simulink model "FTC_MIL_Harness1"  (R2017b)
settings: Solver=FixedStepDiscrete  StartTime=0.0  StopTime=4  FixedStep=0.01  RelTol=1e-3  EnableMultiTasking=on
undefined symbols (not defined in the file): sigbuilder_block

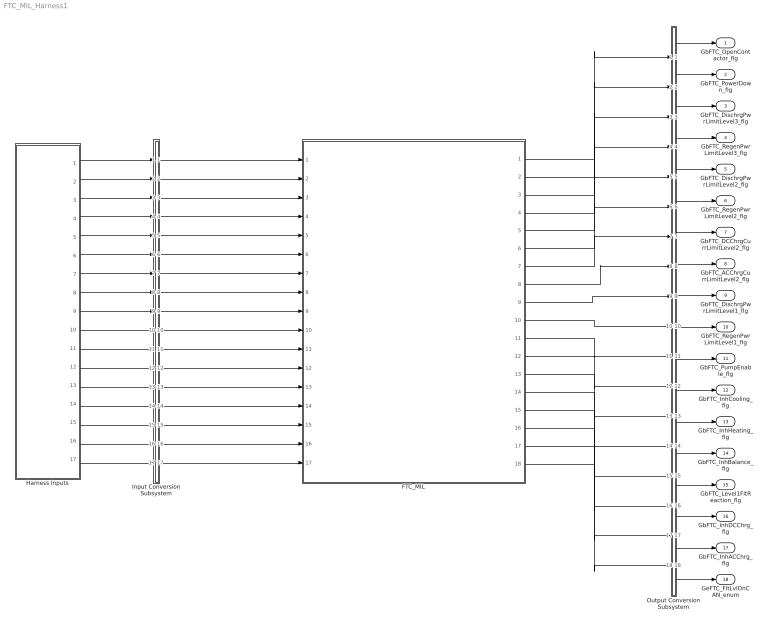
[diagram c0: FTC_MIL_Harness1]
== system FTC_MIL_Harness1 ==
  FTC_MIL : ModelReference  ModelNameDialog=FTC_MIL  SimulationMode=Normal  ModelReferenceVersion='M102C103'
  Harness Inputs : Subsystem  Tag=STV Subsys  LoadFcn=sigbuilder_block('load');  StartFcn=sigbuilder_block('start');  StopFcn=sigbuilder_block('stop');  ClipboardFcn=sigbuilder_block('clipboard');  mask(Sigbuilder block){tuvar=[0:10]}
      mask init:
      | if ~strcmp(get_param(bdroot(gcb),'SimulationStatus'),'stopped'),tuvar = sigbuilder_block('maskInit'); end
  Input Conversion Subsystem : Subsystem  Tag=__SLT_ICS__  Description=Signal spec. and routing
  Output Conversion Subsystem : Subsystem  Tag=__SLT_OCS__  Description=Signal spec. and routing
  GbFTC_OpenContactor_flg : Outport  OutDataTypeStr=boolean  PortDimensions=[1]
  GbFTC_PowerDown_flg : Outport  Port=2  OutDataTypeStr=boolean  PortDimensions=[1]
  GbFTC_DischrgPwrLimitLevel3_flg : Outport  Port=3  OutDataTypeStr=boolean  PortDimensions=[1]
  GbFTC_RegenPwrLimitLevel3_flg : Outport  Port=4  OutDataTypeStr=boolean  PortDimensions=[1]
  GbFTC_DischrgPwrLimitLevel2_flg : Outport  Port=5  OutDataTypeStr=boolean  PortDimensions=[1]
  GbFTC_RegenPwrLimitLevel2_flg : Outport  Port=6  OutDataTypeStr=boolean  PortDimensions=[1]
  GbFTC_DCChrgCurrLimitLevel2_flg : Outport  Port=7  OutDataTypeStr=boolean  PortDimensions=[1]
  GbFTC_ACChrgCurrLimitLevel2_flg : Outport  Port=8  OutDataTypeStr=boolean  PortDimensions=[1]
  GbFTC_DischrgPwrLimitLevel1_flg : Outport  Port=9  OutDataTypeStr=boolean  PortDimensions=[1]
  GbFTC_RegenPwrLimitLevel1_flg : Outport  Port=10  OutDataTypeStr=boolean  PortDimensions=[1]
  GbFTC_PumpEnable_flg : Outport  Port=11  OutDataTypeStr=boolean  PortDimensions=[1]
  GbFTC_InhCooling_flg : Outport  Port=12  OutDataTypeStr=boolean  PortDimensions=[1]
  GbFTC_InhHeating_flg : Outport  Port=13  OutDataTypeStr=boolean  PortDimensions=[1]
  GbFTC_InhBalance_flg : Outport  Port=14  OutDataTypeStr=boolean  PortDimensions=[1]
  GbFTC_Level1FltReaction_flg : Outport  Port=15  OutDataTypeStr=boolean  PortDimensions=[1]
  GbFTC_InhDCChrg_flg : Outport  Port=16  OutDataTypeStr=boolean  PortDimensions=[1]
  GbFTC_InhACChrg_flg : Outport  Port=17  OutDataTypeStr=boolean  PortDimensions=[1]
  GeFTC_FltLvlOnCAN_enum : Outport  Port=18  OutDataTypeStr=uint8  PortDimensions=[1]
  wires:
  Harness Inputs/1(GbISP_OpenContactor_flg) -> Input Conversion Subsystem/1(Inport_1)
  Harness Inputs/2(GbISP_PowerDown_flg) -> Input Conversion Subsystem/2(Inport_2)
  Harness Inputs/3(GbISP_DischrgPwrLimitLevel3_flg) -> Input Conversion Subsystem/3(Inport_3)
  Harness Inputs/4(GbISP_RegenPwrLimitLevel3_flg) -> Input Conversion Subsystem/4(Inport_4)
  Harness Inputs/5(GbISP_DischrgPwrLimitLevel2_flg) -> Input Conversion Subsystem/5(Inport_5)
  Harness Inputs/6(GbISP_RegenPwrLimitLevel2_flg) -> Input Conversion Subsystem/6(Inport_6)
  Harness Inputs/7(GbISP_DCChrgCurrLimitLevel2_flg) -> Input Conversion Subsystem/7(Inport_7)
  Harness Inputs/8(GbISP_ACChrgCurrLimitLevel2_flg) -> Input Conversion Subsystem/8(Inport_8)
  Harness Inputs/9(GbISP_DischrgPwrLimitLevel1_flg) -> Input Conversion Subsystem/9(Inport_9)
  Harness Inputs/10(GbISP_RegenPwrLimitLevel1_flg) -> Input Conversion Subsystem/10(Inport_10)
  Harness Inputs/11(GbISP_PumpEnable_flg) -> Input Conversion Subsystem/11(Inport_11)
  Harness Inputs/12(GbISP_InhCooling_flg) -> Input Conversion Subsystem/12(Inport_12)
  Harness Inputs/13(GbISP_InhHeating_flg) -> Input Conversion Subsystem/13(Inport_13)
  Harness Inputs/14(GbISP_InhBalance_flg) -> Input Conversion Subsystem/14(Inport_14)
  Harness Inputs/15(GbISP_FltReactionReserved_flg) -> Input Conversion Subsystem/15(Inport_15)
  Harness Inputs/16(GbISP_InhDCChrg_flg) -> Input Conversion Subsystem/16(Inport_16)
  Harness Inputs/17(GbISP_InhACChrg_flg) -> Input Conversion Subsystem/17(Inport_17)
  Output Conversion Subsystem/1(Outport_1) -> GbFTC_OpenContactor_flg/1
  Output Conversion Subsystem/2(Outport_2) -> GbFTC_PowerDown_flg/1
  Output Conversion Subsystem/3(Outport_3) -> GbFTC_DischrgPwrLimitLevel3_flg/1
  Output Conversion Subsystem/4(Outport_4) -> GbFTC_RegenPwrLimitLevel3_flg/1
  Output Conversion Subsystem/5(Outport_5) -> GbFTC_DischrgPwrLimitLevel2_flg/1
  Output Conversion Subsystem/6(Outport_6) -> GbFTC_RegenPwrLimitLevel2_flg/1
  Output Conversion Subsystem/7(Outport_7) -> GbFTC_DCChrgCurrLimitLevel2_flg/1
  Output Conversion Subsystem/8(Outport_8) -> GbFTC_ACChrgCurrLimitLevel2_flg/1
  Output Conversion Subsystem/9(Outport_9) -> GbFTC_DischrgPwrLimitLevel1_flg/1
  Output Conversion Subsystem/10(Outport_10) -> GbFTC_RegenPwrLimitLevel1_flg/1
  Output Conversion Subsystem/11(Outport_11) -> GbFTC_PumpEnable_flg/1
  Output Conversion Subsystem/12(Outport_12) -> GbFTC_InhCooling_flg/1
  Output Conversion Subsystem/13(Outport_13) -> GbFTC_InhHeating_flg/1
  Output Conversion Subsystem/14(Outport_14) -> GbFTC_InhBalance_flg/1
  Output Conversion Subsystem/15(Outport_15) -> GbFTC_Level1FltReaction_flg/1
  Output Conversion Subsystem/16(Outport_16) -> GbFTC_InhDCChrg_flg/1
  Output Conversion Subsystem/17(Outport_17) -> GbFTC_InhACChrg_flg/1
  Output Conversion Subsystem/18(Outport_18) -> GeFTC_FltLvlOnCAN_enum/1
  Input Conversion Subsystem/1(Outport_1) -> FTC_MIL/1
  Input Conversion Subsystem/2(Outport_2) -> FTC_MIL/2
  Input Conversion Subsystem/3(Outport_3) -> FTC_MIL/3
  Input Conversion Subsystem/4(Outport_4) -> FTC_MIL/4
  Input Conversion Subsystem/5(Outport_5) -> FTC_MIL/5
  Input Conversion Subsystem/6(Outport_6) -> FTC_MIL/6
  Input Conversion Subsystem/7(Outport_7) -> FTC_MIL/7
  Input Conversion Subsystem/8(Outport_8) -> FTC_MIL/8
  Input Conversion Subsystem/9(Outport_9) -> FTC_MIL/9
  Input Conversion Subsystem/10(Outport_10) -> FTC_MIL/10
  Input Conversion Subsystem/11(Outport_11) -> FTC_MIL/11
  Input Conversion Subsystem/12(Outport_12) -> FTC_MIL/12
  Input Conversion Subsystem/13(Outport_13) -> FTC_MIL/13
  Input Conversion Subsystem/14(Outport_14) -> FTC_MIL/14
  Input Conversion Subsystem/15(Outport_15) -> FTC_MIL/15
  Input Conversion Subsystem/16(Outport_16) -> FTC_MIL/16
  Input Conversion Subsystem/17(Outport_17) -> FTC_MIL/17
  FTC_MIL/1 -> Output Conversion Subsystem/1(Inport_1)
  FTC_MIL/2 -> Output Conversion Subsystem/2(Inport_2)
  FTC_MIL/3 -> Output Conversion Subsystem/3(Inport_3)
  FTC_MIL/4 -> Output Conversion Subsystem/4(Inport_4)
  FTC_MIL/5 -> Output Conversion Subsystem/5(Inport_5)
  FTC_MIL/6 -> Output Conversion Subsystem/6(Inport_6)
  FTC_MIL/7 -> Output Conversion Subsystem/7(Inport_7)
  FTC_MIL/8 -> Output Conversion Subsystem/8(Inport_8)
  FTC_MIL/9 -> Output Conversion Subsystem/9(Inport_9)
  FTC_MIL/10 -> Output Conversion Subsystem/10(Inport_10)
  FTC_MIL/11 -> Output Conversion Subsystem/11(Inport_11)
  FTC_MIL/12 -> Output Conversion Subsystem/12(Inport_12)
  FTC_MIL/13 -> Output Conversion Subsystem/13(Inport_13)
  FTC_MIL/14 -> Output Conversion Subsystem/14(Inport_14)
  FTC_MIL/15 -> Output Conversion Subsystem/15(Inport_15)
  FTC_MIL/16 -> Output Conversion Subsystem/16(Inport_16)
  FTC_MIL/17 -> Output Conversion Subsystem/17(Inport_17)
  FTC_MIL/18 -> Output Conversion Subsystem/18(Inport_18)

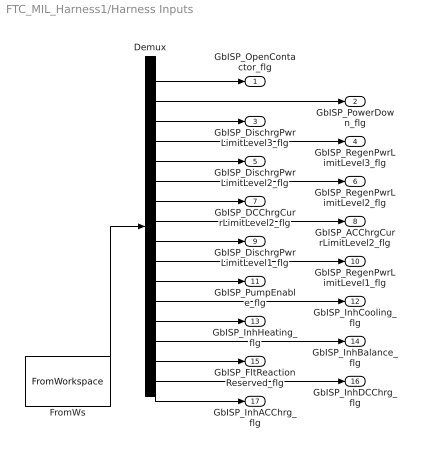
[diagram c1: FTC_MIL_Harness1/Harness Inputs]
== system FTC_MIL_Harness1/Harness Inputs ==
  Demux : Demux  Tag=STV Demux  Outputs=17
  FromWs : FromWorkspace  Tag=STV FromWs  VariableName=tuvar  SampleTime=0
  GbISP_OpenContactor_flg : Outport  Tag=STV Outport
  GbISP_PowerDown_flg : Outport  Tag=STV Outport  Port=2
  GbISP_DischrgPwrLimitLevel3_flg : Outport  Tag=STV Outport  Port=3
  GbISP_RegenPwrLimitLevel3_flg : Outport  Tag=STV Outport  Port=4
  GbISP_DischrgPwrLimitLevel2_flg : Outport  Tag=STV Outport  Port=5
  GbISP_RegenPwrLimitLevel2_flg : Outport  Tag=STV Outport  Port=6
  GbISP_DCChrgCurrLimitLevel2_flg : Outport  Tag=STV Outport  Port=7
  GbISP_ACChrgCurrLimitLevel2_flg : Outport  Tag=STV Outport  Port=8
  GbISP_DischrgPwrLimitLevel1_flg : Outport  Tag=STV Outport  Port=9
  GbISP_RegenPwrLimitLevel1_flg : Outport  Tag=STV Outport  Port=10
  GbISP_PumpEnable_flg : Outport  Tag=STV Outport  Port=11
  GbISP_InhCooling_flg : Outport  Tag=STV Outport  Port=12
  GbISP_InhHeating_flg : Outport  Tag=STV Outport  Port=13
  GbISP_InhBalance_flg : Outport  Tag=STV Outport  Port=14
  GbISP_FltReactionReserved_flg : Outport  Tag=STV Outport  Port=15
  GbISP_InhDCChrg_flg : Outport  Tag=STV Outport  Port=16
  GbISP_InhACChrg_flg : Outport  Tag=STV Outport  Port=17
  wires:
  FromWs/1 -> Demux/1
  Demux/1 -> GbISP_OpenContactor_flg/1
  Demux/2 -> GbISP_PowerDown_flg/1
  Demux/3 -> GbISP_DischrgPwrLimitLevel3_flg/1
  Demux/4 -> GbISP_RegenPwrLimitLevel3_flg/1
  Demux/5 -> GbISP_DischrgPwrLimitLevel2_flg/1
  Demux/6 -> GbISP_RegenPwrLimitLevel2_flg/1
  Demux/7 -> GbISP_DCChrgCurrLimitLevel2_flg/1
  Demux/8 -> GbISP_ACChrgCurrLimitLevel2_flg/1
  Demux/9 -> GbISP_DischrgPwrLimitLevel1_flg/1
  Demux/10 -> GbISP_RegenPwrLimitLevel1_flg/1
  Demux/11 -> GbISP_PumpEnable_flg/1
  Demux/12 -> GbISP_InhCooling_flg/1
  Demux/13 -> GbISP_InhHeating_flg/1
  Demux/14 -> GbISP_InhBalance_flg/1
  Demux/15 -> GbISP_FltReactionReserved_flg/1
  Demux/16 -> GbISP_InhDCChrg_flg/1
  Demux/17 -> GbISP_InhACChrg_flg/1

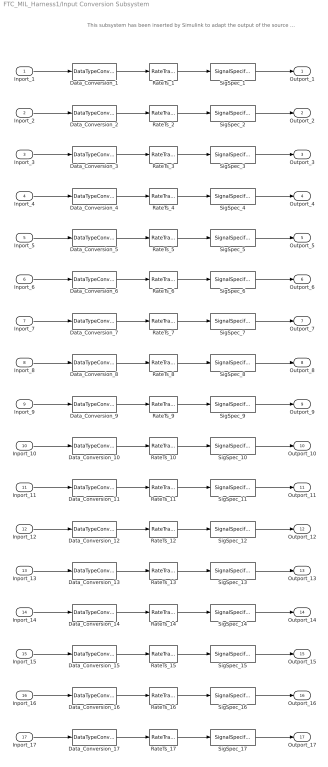
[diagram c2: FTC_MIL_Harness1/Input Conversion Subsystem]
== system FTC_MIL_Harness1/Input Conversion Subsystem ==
  note: This subsystem has been inserted by Simulink to adapt the output of the source blocks to the interface required by the harnessed component. Modifying the contents of this subsystem may result in compilation and simulation failure.
  Inport_1 : Inport
  Inport_2 : Inport  Port=2
  Inport_3 : Inport  Port=3
  Inport_4 : Inport  Port=4
  Inport_5 : Inport  Port=5
  Inport_6 : Inport  Port=6
  Inport_7 : Inport  Port=7
  Inport_8 : Inport  Port=8
  Inport_9 : Inport  Port=9
  Inport_10 : Inport  Port=10
  Inport_11 : Inport  Port=11
  Inport_12 : Inport  Port=12
  Inport_13 : Inport  Port=13
  Inport_14 : Inport  Port=14
  Inport_15 : Inport  Port=15
  Inport_16 : Inport  Port=16
  Inport_17 : Inport  Port=17
  Data_Conversion_{1..17} (17 alike) : DataTypeConversion  OutDataTypeStr=boolean
  RateTs_{1..17} (17 alike) : RateTransition  OutPortSampleTime=0.01
  SigSpec_{1..17} (17 alike) : SignalSpecification  OutDataTypeStr=boolean  Unit=flag  Dimensions=[1]  SampleTime=0.01
  Outport_1 : Outport
  Outport_2 : Outport  Port=2
  Outport_3 : Outport  Port=3
  Outport_4 : Outport  Port=4
  Outport_5 : Outport  Port=5
  Outport_6 : Outport  Port=6
  Outport_7 : Outport  Port=7
  Outport_8 : Outport  Port=8
  Outport_9 : Outport  Port=9
  Outport_10 : Outport  Port=10
  Outport_11 : Outport  Port=11
  Outport_12 : Outport  Port=12
  Outport_13 : Outport  Port=13
  Outport_14 : Outport  Port=14
  Outport_15 : Outport  Port=15
  Outport_16 : Outport  Port=16
  Outport_17 : Outport  Port=17
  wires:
  SigSpec_1/1 -> Outport_1/1
  RateTs_1/1 -> SigSpec_1/1
  Data_Conversion_1/1 -> RateTs_1/1
  Inport_1/1 -> Data_Conversion_1/1
  SigSpec_2/1 -> Outport_2/1
  RateTs_2/1 -> SigSpec_2/1
  Data_Conversion_2/1 -> RateTs_2/1
  Inport_2/1 -> Data_Conversion_2/1
  SigSpec_3/1 -> Outport_3/1
  RateTs_3/1 -> SigSpec_3/1
  Data_Conversion_3/1 -> RateTs_3/1
  Inport_3/1 -> Data_Conversion_3/1
  SigSpec_4/1 -> Outport_4/1
  RateTs_4/1 -> SigSpec_4/1
  Data_Conversion_4/1 -> RateTs_4/1
  Inport_4/1 -> Data_Conversion_4/1
  SigSpec_5/1 -> Outport_5/1
  RateTs_5/1 -> SigSpec_5/1
  Data_Conversion_5/1 -> RateTs_5/1
  Inport_5/1 -> Data_Conversion_5/1
  SigSpec_6/1 -> Outport_6/1
  RateTs_6/1 -> SigSpec_6/1
  Data_Conversion_6/1 -> RateTs_6/1
  Inport_6/1 -> Data_Conversion_6/1
  SigSpec_7/1 -> Outport_7/1
  RateTs_7/1 -> SigSpec_7/1
  Data_Conversion_7/1 -> RateTs_7/1
  Inport_7/1 -> Data_Conversion_7/1
  SigSpec_8/1 -> Outport_8/1
  RateTs_8/1 -> SigSpec_8/1
  Data_Conversion_8/1 -> RateTs_8/1
  Inport_8/1 -> Data_Conversion_8/1
  SigSpec_9/1 -> Outport_9/1
  RateTs_9/1 -> SigSpec_9/1
  Data_Conversion_9/1 -> RateTs_9/1
  Inport_9/1 -> Data_Conversion_9/1
  SigSpec_10/1 -> Outport_10/1
  RateTs_10/1 -> SigSpec_10/1
  Data_Conversion_10/1 -> RateTs_10/1
  Inport_10/1 -> Data_Conversion_10/1
  SigSpec_11/1 -> Outport_11/1
  RateTs_11/1 -> SigSpec_11/1
  Data_Conversion_11/1 -> RateTs_11/1
  Inport_11/1 -> Data_Conversion_11/1
  SigSpec_12/1 -> Outport_12/1
  RateTs_12/1 -> SigSpec_12/1
  Data_Conversion_12/1 -> RateTs_12/1
  Inport_12/1 -> Data_Conversion_12/1
  SigSpec_13/1 -> Outport_13/1
  RateTs_13/1 -> SigSpec_13/1
  Data_Conversion_13/1 -> RateTs_13/1
  Inport_13/1 -> Data_Conversion_13/1
  SigSpec_14/1 -> Outport_14/1
  RateTs_14/1 -> SigSpec_14/1
  Data_Conversion_14/1 -> RateTs_14/1
  Inport_14/1 -> Data_Conversion_14/1
  SigSpec_15/1 -> Outport_15/1
  RateTs_15/1 -> SigSpec_15/1
  Data_Conversion_15/1 -> RateTs_15/1
  Inport_15/1 -> Data_Conversion_15/1
  SigSpec_16/1 -> Outport_16/1
  RateTs_16/1 -> SigSpec_16/1
  Data_Conversion_16/1 -> RateTs_16/1
  Inport_16/1 -> Data_Conversion_16/1
  SigSpec_17/1 -> Outport_17/1
  RateTs_17/1 -> SigSpec_17/1
  Data_Conversion_17/1 -> RateTs_17/1
  Inport_17/1 -> Data_Conversion_17/1

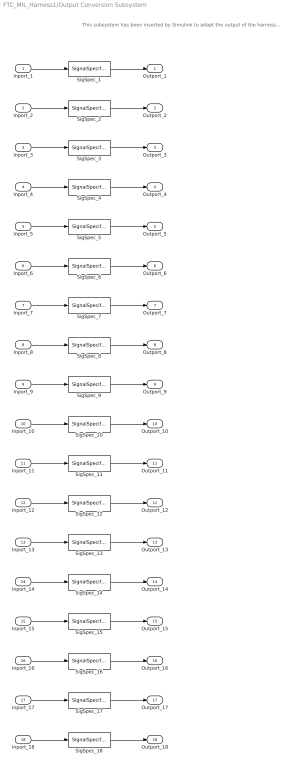
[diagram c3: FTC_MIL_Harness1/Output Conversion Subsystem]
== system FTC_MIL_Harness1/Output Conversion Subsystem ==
  note: This subsystem has been inserted by Simulink to adapt the output of the harnessed component to the interface required by the sink blocks. Modifying the contents of this subsystem may result in compilation and simulation failure.
  Inport_1 : Inport
  Inport_2 : Inport  Port=2
  Inport_3 : Inport  Port=3
  Inport_4 : Inport  Port=4
  Inport_5 : Inport  Port=5
  Inport_6 : Inport  Port=6
  Inport_7 : Inport  Port=7
  Inport_8 : Inport  Port=8
  Inport_9 : Inport  Port=9
  Inport_10 : Inport  Port=10
  Inport_11 : Inport  Port=11
  Inport_12 : Inport  Port=12
  Inport_13 : Inport  Port=13
  Inport_14 : Inport  Port=14
  Inport_15 : Inport  Port=15
  Inport_16 : Inport  Port=16
  Inport_17 : Inport  Port=17
  Inport_18 : Inport  Port=18
  SigSpec_{1..17} (17 alike) : SignalSpecification  OutDataTypeStr=boolean  Unit=flag  Dimensions=[1]  SampleTime=0.01
  SigSpec_18 : SignalSpecification  OutDataTypeStr=uint8  Unit=enum  Dimensions=[1]  SampleTime=0.01
  Outport_1 : Outport
  Outport_2 : Outport  Port=2
  Outport_3 : Outport  Port=3
  Outport_4 : Outport  Port=4
  Outport_5 : Outport  Port=5
  Outport_6 : Outport  Port=6
  Outport_7 : Outport  Port=7
  Outport_8 : Outport  Port=8
  Outport_9 : Outport  Port=9
  Outport_10 : Outport  Port=10
  Outport_11 : Outport  Port=11
  Outport_12 : Outport  Port=12
  Outport_13 : Outport  Port=13
  Outport_14 : Outport  Port=14
  Outport_15 : Outport  Port=15
  Outport_16 : Outport  Port=16
  Outport_17 : Outport  Port=17
  Outport_18 : Outport  Port=18
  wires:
  Inport_1/1 -> SigSpec_1/1
  SigSpec_1/1 -> Outport_1/1
  Inport_2/1 -> SigSpec_2/1
  SigSpec_2/1 -> Outport_2/1
  Inport_3/1 -> SigSpec_3/1
  SigSpec_3/1 -> Outport_3/1
  Inport_4/1 -> SigSpec_4/1
  SigSpec_4/1 -> Outport_4/1
  Inport_5/1 -> SigSpec_5/1
  SigSpec_5/1 -> Outport_5/1
  Inport_6/1 -> SigSpec_6/1
  SigSpec_6/1 -> Outport_6/1
  Inport_7/1 -> SigSpec_7/1
  SigSpec_7/1 -> Outport_7/1
  Inport_8/1 -> SigSpec_8/1
  SigSpec_8/1 -> Outport_8/1
  Inport_9/1 -> SigSpec_9/1
  SigSpec_9/1 -> Outport_9/1
  Inport_10/1 -> SigSpec_10/1
  SigSpec_10/1 -> Outport_10/1
  Inport_11/1 -> SigSpec_11/1
  SigSpec_11/1 -> Outport_11/1
  Inport_12/1 -> SigSpec_12/1
  SigSpec_12/1 -> Outport_12/1
  Inport_13/1 -> SigSpec_13/1
  SigSpec_13/1 -> Outport_13/1
  Inport_14/1 -> SigSpec_14/1
  SigSpec_14/1 -> Outport_14/1
  Inport_15/1 -> SigSpec_15/1
  SigSpec_15/1 -> Outport_15/1
  Inport_16/1 -> SigSpec_16/1
  SigSpec_16/1 -> Outport_16/1
  Inport_17/1 -> SigSpec_17/1
  SigSpec_17/1 -> Outport_17/1
  Inport_18/1 -> SigSpec_18/1
  SigSpec_18/1 -> Outport_18/1
